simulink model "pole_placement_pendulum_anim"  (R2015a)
settings: Solver=ode45  StartTime=0.0  StopTime=inf  RelTol=1e-3
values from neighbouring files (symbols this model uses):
  g = 9.81    [pendulum_sys_init.m]
  kc = 2    [pendulum_sys_init.m]
  ke = 2    [pendulum_sys_init.m]
  l = 1    [pendulum_sys_init.m]
  M = 10    [pendulum_sys_init.m]
  m = 2    [pendulum_sys_init.m]
  ra = 10    [pendulum_sys_init.m]
  rr = .1    (= 0.1)    [pendulum_sys_init.m]
undefined symbols (not defined in the file or in its folder): K, pendolo_sys_diff
libraries: vrlib x1

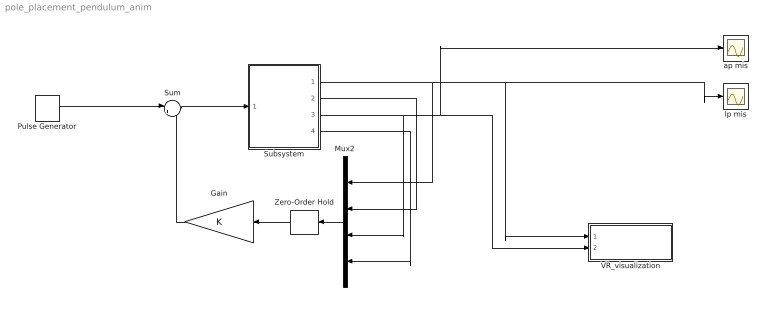
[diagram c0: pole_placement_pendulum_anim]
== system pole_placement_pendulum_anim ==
  Gain : Gain  Gain=K  Multiplication=Matrix(K*u)
  Mux2 : Mux
  Pulse Generator : DiscretePulseGenerator  PulseType=Time based  Amplitude=5  Period=5  PulseWidth=50
  Subsystem : Subsystem
  Sum : Sum  Inputs=|+-
  VR_visualization : Subsystem
  Zero-Order Hold : ZeroOrderHold  SampleTime=0.1
  ap mis : Scope
  lp mis : Scope
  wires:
  Subsystem/1(lp) -> Mux2/1, lp mis/1, VR_visualization/1(lp)
  Pulse Generator/1 -> Sum/1
  Subsystem/3(ap) -> Mux2/3, ap mis/1, VR_visualization/2(ap)
  Subsystem/2(lv) -> Mux2/2
  Subsystem/4(av) -> Mux2/4
  Sum/1 -> Subsystem/1(voltage)
  Gain/1 -> Sum/2
  Zero-Order Hold/1 -> Gain/1
  Mux2/1 -> Zero-Order Hold/1

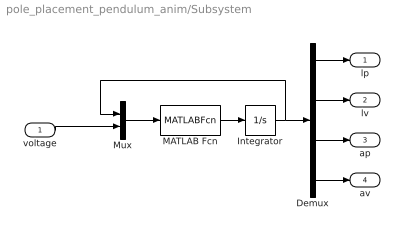
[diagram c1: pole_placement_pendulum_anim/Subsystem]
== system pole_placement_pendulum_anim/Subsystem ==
  voltage : Inport
  Demux : Demux
  Integrator : Integrator  InitialCondition=[0 0.0 0.1 0]
  MATLAB Fcn : MATLABFcn  MATLABFcn=pendolo_sys_diff(u,M,m,l,ra,rr,ke,kc,g)
  Mux : Mux  Inputs=2
  lp : Outport
  lv : Outport  Port=2
  ap : Outport  Port=3
  av : Outport  Port=4
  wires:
  MATLAB Fcn/1 -> Integrator/1
  Integrator/1 -> Demux/1, Mux/1
  Demux/4 -> av/1
  Demux/3 -> ap/1
  Demux/2 -> lv/1
  Demux/1 -> lp/1
  Mux/1 -> MATLAB Fcn/1
  voltage/1 -> Mux/2

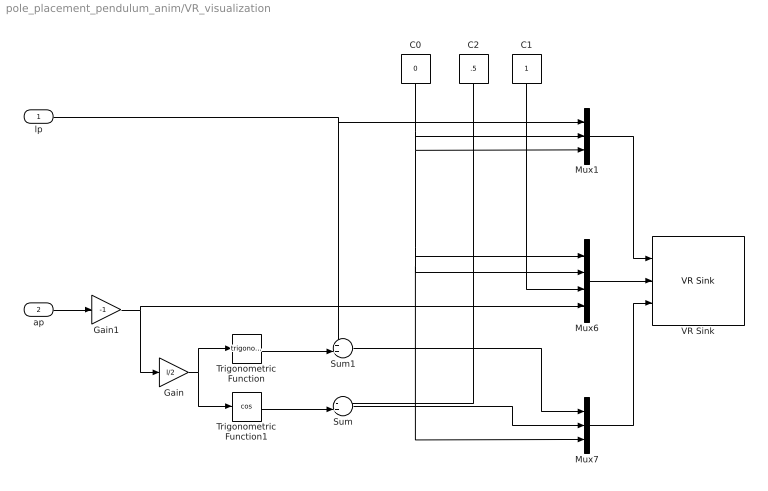
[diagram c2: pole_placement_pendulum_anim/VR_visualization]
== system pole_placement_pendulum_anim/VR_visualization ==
  lp : Inport
  ap : Inport  Port=2
  C0 : Constant  Value=0
  C1 : Constant
  C2 : Constant  Value=.5
  Gain : Gain  Gain=l/2
  Gain1 : Gain  Gain=-1
  Mux1 : Mux  Inputs=3
  Mux6 : Mux
  Mux7 : Mux  Inputs=3
  Sum : Sum  Inputs=-+|
  Sum1 : Sum  Inputs=++|
  Trigonometric Function : Trigonometry
  Trigonometric Function1 : Trigonometry  Operator=cos
  VR Sink : vrlib/VR Sink  InstantiateOnLoad=on  SampleTime=0.02  ViewEnable=on  RemoteChange=off  RemoteView=off  FieldsWritten=carrello.translation.3.1.double#asta.rotation.4.1.double#asta.translation.3.1.double  WorldFileName=vrml1.wrl  AutoView=on  VideoDimensions=[]  AllowVariableSize=off
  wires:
  Mux1/1 -> VR Sink/1
  Mux6/1 -> VR Sink/2
  Mux7/1 -> VR Sink/3
  lp/1 -> Mux1/1, Sum1/1
  C0/1 -> Mux1/2, Mux1/3, Mux6/1, Mux6/2, Mux7/3
  ap/1 -> Gain1/1
  C1/1 -> Mux6/3
  Trigonometric Function/1 -> Sum1/2
  Trigonometric Function1/1 -> Sum/2
  Sum1/1 -> Mux7/1
  Sum/1 -> Mux7/2
  C2/1 -> Sum/1
  Gain/1 -> Trigonometric Function/1, Trigonometric Function1/1
  Gain1/1 -> Mux6/4, Gain/1
